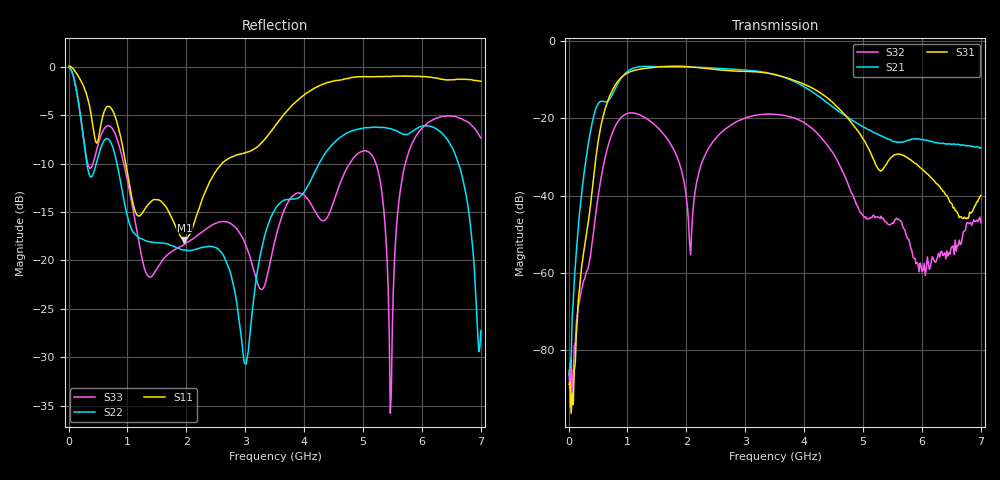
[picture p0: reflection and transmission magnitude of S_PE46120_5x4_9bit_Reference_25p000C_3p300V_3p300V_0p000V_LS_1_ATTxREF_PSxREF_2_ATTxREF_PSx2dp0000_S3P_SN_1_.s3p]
! Device ID: PE46120_5x4_9bit_Reference
! Device ID: PE46120_5x4_9bit_Reference
! File Path: z:\PE46120_5x4_9bit_Reference\MPAC_Yi\new_12port\25p000C\3p300\LS_1_ATTxREF_PSxREF_2_ATTxREF_PSx2dp0000\PE46120_5x4_9bit_Reference_25p000C_3p300V_3p300V_0p000V_LS_1_ATTxREF_PSxREF_2_ATTxREF_PSx2dp0000_S3P_SN_1_.s3p
! Serial: 1
! Lot:
! Temp: 25.000C
! VDD: 3.300
! VSS: 0.000
! Control_Hi: 3.300
! Control_Lo: 0.000
! Logic State: LS_1_ATTxREF_PSxREF_2_ATTxREF_PSx2dp0000
! Port 1: RFin
! Port 2: RFout1
! Port 3: RFout2
! ThroughPath:1-3
! IDD: -0.0005392795
! ISS: 0
! Comment:
#  Hz  S  RI  R  50
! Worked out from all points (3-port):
!   401 points, 10 MHz to 7 GHz, reference 50 ohm
!   strongest paths, dB at 10 MHz, 1.758 GHz, 3.505 GHz, 5.253 GHz, 7 GHz:
!     S31: -88.8, -6.5, -8.7, -33.0, -39.9
!     S21: -86.5, -6.7, -8.6, -24.1, -27.6
!     S32: -85.2, -27.3, -18.9, -45.5, -47.0
!   lowest |S11| = -17.9 dB at 1.967 GHz (marker M1), VSWR 1.29, Z = 62.1 + j7.68 ohm
!   |S11| at or under -10 dB: 971.7 MHz to 2.604 GHz (1.632 GHz wide, 91.3 % of centre)
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1e7  1.001 -0.1151  -5.64e-05 -5.44e-05  -9.01e-05 2.57e-05
     -1.61e-05 -4.47e-05  0.9872 -0.0963  1.01e-05 -0.000114
     3.55e-05 6.73e-06  -1.38e-05 5.32e-05  0.9877 -0.0964
2.5465e8  -0.5338 -0.5878  -0.0161 -0.00582  -0.000383 -0.00168
          -0.0161 -0.00593  -0.3288 -0.2681  -0.000288 0.000623
          -0.00036 -0.00176  -0.000282 0.000743  -0.3368 -0.2664
4.81825e8  -0.3929 -0.0895  -0.0461 0.1352  -0.0172 -0.0345
           -0.0464 0.137  0.1908 0.2641  0.00701 0.00238
           -0.0174 -0.0349  0.00705 0.00242  0.1905 0.3247
1.02355e9  -0.1152 0.2291  0.367 -0.1892  0.3466 0.1792
           0.3711 -0.1923  -0.0465 -0.1518  0.1015 0.0557
           0.3511 0.1808  0.1029 0.0562  -0.1229 -0.2034
1.9672e9  0.112 0.0608  -0.3839 0.2483  -0.4577 -0.0831
          -0.3883 0.2517  -0.0952 0.0612  0.0062 0.0125
          -0.463 -0.0831  0.00646 0.0127  -0.1208 0.00784
3.505e9  -0.3745 -0.3228  -0.0684 -0.3581  0.2386 -0.2752
         -0.0699 -0.3632  0.0558 0.1744  -0.0891 -0.0669
         0.2409 -0.2789  -0.0906 -0.0676  -0.1266 0.00667
5.1127e9  -0.8338 0.3052  0.0498 0.0483  0.0157 0.034
          0.0511 0.0486  -0.0565 0.4822  0.00473 -0.00168
          0.0162 0.0345  0.0045 -0.00239  0.0336 0.3577
5.479675e9  -0.7383 0.5021  0.0492 0.0155  0.0023 0.0311
            0.0498 0.0152  0.2742 0.3914  0.00373 -0.00196
            0.00197 0.0313  0.00393 -0.00174  -0.0197 -0.00632
5.9515e9  -0.5436 0.7085  0.0507 -0.0163  0.0215 0.00915
          0.0516 -0.0165  0.4668 0.1416  0.000376 -0.000359
          0.0221 0.00927  0.000678 -0.000778  0.156 0.4356
7e9  -0.09 0.8373  -0.0221 -0.0346  0.00529 0.00844
     -0.0232 -0.0348  -0.039 0.0191  -0.003 0.00332
     0.00522 0.00864  -0.00327 0.00304  0.4194 -0.0867
